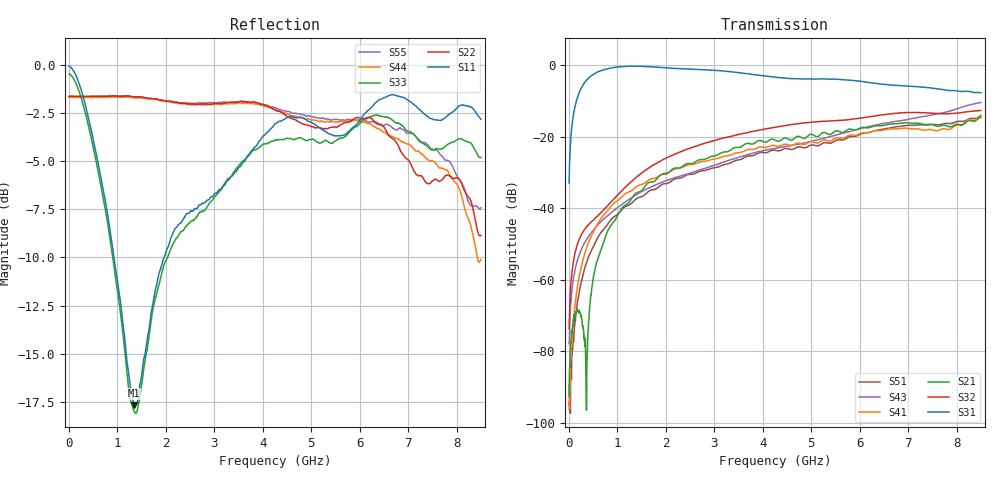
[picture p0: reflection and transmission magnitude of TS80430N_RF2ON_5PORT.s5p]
!Created with skrf (http://scikit-rf.org).
# GHz S RI R 50.0
!freq ReS11 ImS11 ReS12 ImS12 ReS13 ImS13
! ReS14 ImS14 ReS15 ImS15
! ReS21 ImS21 ReS22 ImS22 ReS23 ImS23
! ReS24 ImS24 ReS25 ImS25
! ReS31 ImS31 ReS32 ImS32 ReS33 ImS33
! ReS34 ImS34 ReS35 ImS35
! ReS41 ImS41 ReS42 ImS42 ReS43 ImS43
! ReS44 ImS44 ReS45 ImS45
! ReS51 ImS51 ReS52 ImS52 ReS53 ImS53
! ReS54 ImS54 ReS55 ImS55
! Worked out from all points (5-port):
!   1601 points, 10 MHz to 8.5 GHz, reference 50 ohm
!   strongest paths, dB at 10 MHz, 2.132 GHz, 4.255 GHz, 6.378 GHz, 8.5 GHz:
!     S31: -33.0, -0.9, -3.4, -5.2, -7.8
!     S32: -73.6, -25.2, -17.4, -14.1, -12.7
!     S21: -92.5, -29.2, -21.0, -17.0, -14.6
!     S41: -89.4, -29.5, -22.5, -18.4, -14.1
!     S43: -77.9, -31.7, -23.3, -16.7, -10.5
!     S51: -95.0, -32.3, -23.9, -18.2, -14.2
!   lowest |S11| = -17.7 dB at 1.352 GHz (marker M1), VSWR 1.30, Z = 39.1 + j4.09 ohm
!   |S11| at or under -10 dB: 935.3 MHz to 1.966 GHz (1.031 GHz wide, 71.1 % of centre)
